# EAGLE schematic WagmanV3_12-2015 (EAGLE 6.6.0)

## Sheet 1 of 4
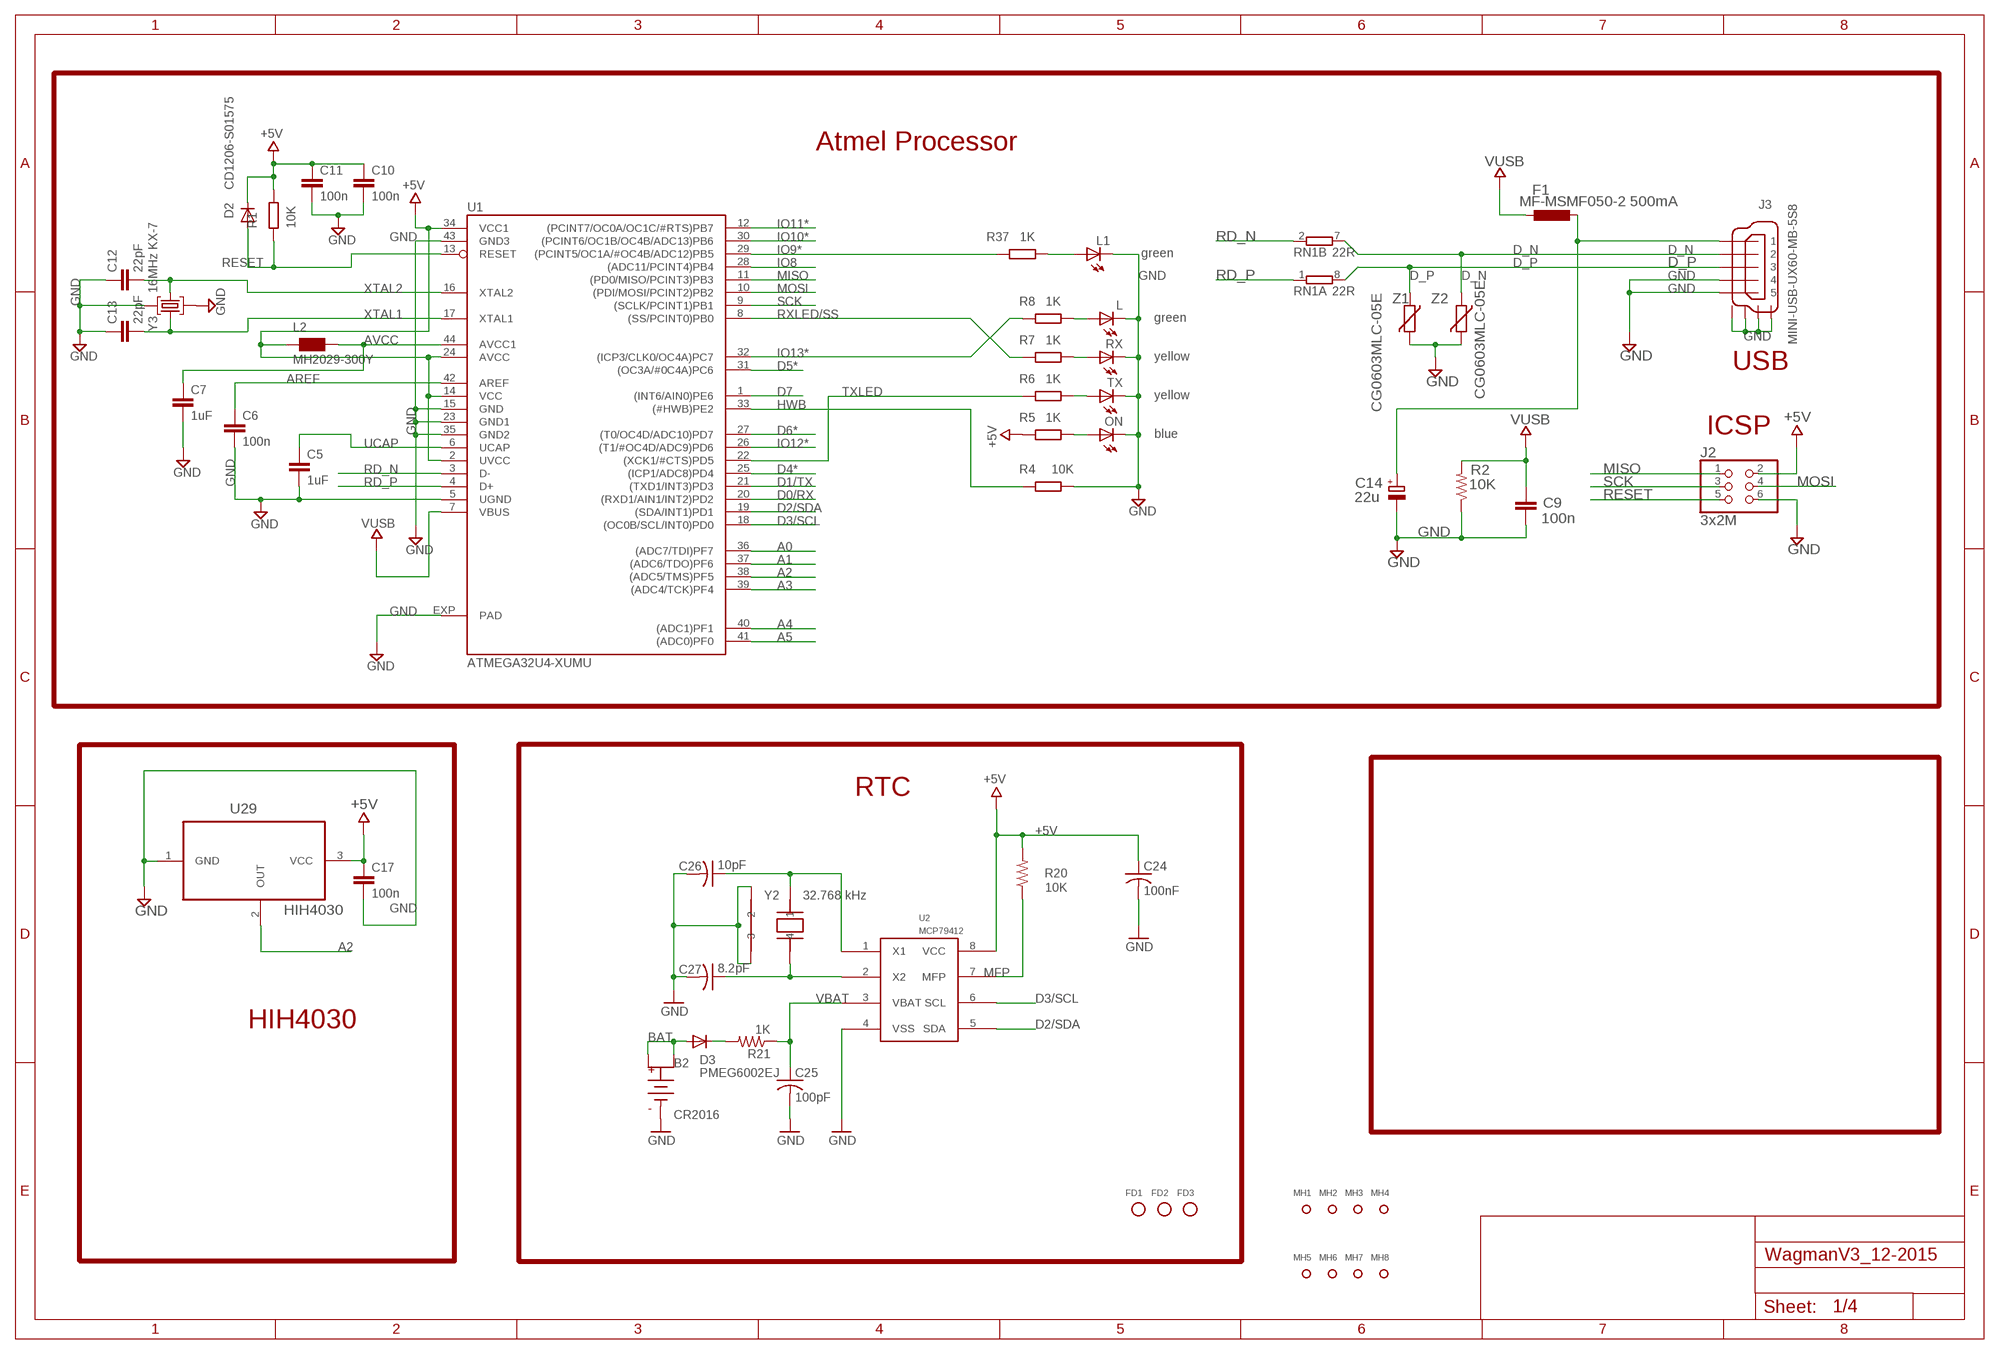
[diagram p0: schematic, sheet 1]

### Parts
B2  CR2016  COIN-CELL-2016-SMT  [BAT-HLD-002-SMT]
C5  1uF  C-EUC0402  [C0402]
C6  100n  C-EUC0402  [C0402]
C7  1uF  C-EUC0402  [C0402]
C9  100n  C-EU0805  [0805]
C10  100n  C-EUC0402  [C0402]
C11  100n  C-EUC0402  [C0402]
C12  22pF  C-EUC0402  [C0402]
C13  22pF  C-EUC0402  [C0402]
C14  22u  CPOL-EUSMCB  [SMC_B]
C17  100n  C-EUC0402  [C0402]
C24  100nF  C-USM0805  [M0805]
C25  100pF  C-USM0805  [M0805]
C26  10pF  C-USM0805  [M0805]
C27  8.2pF  C-USM0805  [M0805]
D2  CD1206-S01575  DIODE-MINIMELF  [MINIMELF]
D3  PMEG6002EJ  DIODESOD-323F  [SOD-323F]
F1  MF-MSMF050-2 500mA  L-EUL1812  [L1812]
FD1  FIDUCIAL-1MM  [FD-1MM]
FD2  FIDUCIAL-1MM  [FD-1MM]
FD3  FIDUCIAL-1MM  [FD-1MM]
J2  3x2M  PINHD-2X3  [2X03]
J3  MINI-USB-UX60-MB-5S8  [UX60-MB-5S8]
L  green  LEDCHIPLED_0805  [CHIPLED_0805]
L1  green  LEDCHIPLED_0805  [CHIPLED_0805]
L2  MH2029-300Y  WE-CBF_0805  [0805]
MH1  MH-3.964  [MH3.964]
MH2  MH-3.964  [MH3.964]
MH3  MH-3.964  [MH3.964]
MH4  MH-3.964  [MH3.964]
MH5  MH-3.964  [MH3.964]
MH6  MH-3.964  [MH3.964]
MH7  MH-3.964  [MH3.964]
MH8  MH-3.964  [MH3.964]
ON  blue  LEDCHIPLED_0805  [CHIPLED_0805]
R1  10K  R-EU_R0402  [R0402]
R2  10K  RESISTOR0805-RES  [0805]
R4  10K  R-EU_R0402  [R0402]
R5  1K  R-EU_R0402  [R0402]
R6  1K  R-EU_R0402  [R0402]
R7  1K  R-EU_R0402  [R0402]
R8  1K  R-EU_R0402  [R0402]
R20  10K  R-US_M0805  [M0805]
R21  1K  R-US_M0805  [M0805]
R37  1K  R-EU_R0402  [R0402]
RN1  22R  4R-NCAY16  [CAY16]
RX  yellow  LEDCHIPLED_0805  [CHIPLED_0805]
TX  yellow  LEDCHIPLED_0805  [CHIPLED_0805]
U1  ATMEGA32U4-XUMU  [QFN44ML7X7]
U2  MCP79412  MCP7941X-SOIC-8  [SO08]
U29  HIH4030  [HIH4030]
Y2  32.768 kHz  CRYSTAL-CITIZEN-CM2XXC  [CRYSTAL-CITIZEN-CM2XXC]
Y3  16MHz KX-7  CRYSTAL-3.2-2.5  [CRYSTAL-3.2-2.5]
Z1  CG0603MLC-05E  VARISTORCN0603  [CT/CN0603]
Z2  CG0603MLC-05E  VARISTORCN0603  [CT/CN0603]

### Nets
+5V: C10.1 C11.1 C17.1 C24.1 D2.C J2.2 L2.1 R1.1 R5.1 R20.2 U1.2(UVCC) U1.14(VCC) U1.24(AVCC) U1.34(VCC1) U2.8(VCC) U29.3(VCC) ; also sheet 2,3,4
A0: U1.36((ADC7/TDI)PF7) ; also sheet 4
A1: U1.37((ADC6/TDO)PF6) ; also sheet 4
A2: U1.38((ADC5/TMS)PF5) U29.2(OUT)
A3: U1.39((ADC4/TCK)PF4) ; also sheet 4
A4: U1.40((ADC1)PF1) ; also sheet 4
A5: U1.41((ADC0)PF0) ; also sheet 4
AREF: C6.1 U1.42(AREF)
AVCC: C7.1 L2.2 U1.44(AVCC1)
BAT: B2.POS1 B2.POS2 D3.A
D0/RX: U1.20((RXD1/AIN1/INT2)PD2) ; also sheet 3
D1/TX: U1.21((TXD1/INT3)PD3) ; also sheet 3
D2/SDA: U1.19((SDA/INT1)PD1) U2.5(SDA) ; also sheet 3
D3/SCL: U1.18((OC0B/SCL/INT0)PD0) U2.6(SCL) ; also sheet 3
D4*: U1.25((ICP1/ADC8)PD4) ; also sheet 3,4
D5*: U1.31((OC3A/#0C4A)PC6) ; also sheet 3
D6*: U1.27((T0/OC4D/ADC10)PD7) ; also sheet 3,4
D7: U1.1((INT6/AIN0)PE6) ; also sheet 4
D_N: J3.2 RN1.7 Z2.1
D_P: J3.3 RN1.8 Z1.1
GND: B2.NEG(B-) C5.2 C6.2 C7.2 C9.2 C10.2 C11.2 C12.1 C13.1 C14.- C17.2 C24.2 C25.2 C26.2 C27.2 J2.6 J3.4 J3.5 J3.M1 J3.M2 J3.M3 J3.M4 L1.C L.C ON.C R2.1 R4.2 RX.C TX.C U1.5(UGND) U1.15(GND) U1.23(GND1) U1.35(GND2) U1.43(GND3) U1.EXP(PAD) U2.4(VSS) U29.1(GND) Y2.P$2 Y2.P$3 Y3.2(GND) Y3.4(GND) Z1.2 Z2.2 ; also sheet 2,3,4
HWB: R4.1 U1.33((#HWB)PE2)
IO8: U1.28((ADC11/PCINT4)PB4) ; also sheet 3,4
IO9*: R37.1 U1.29((PCINT5/OC1A/#OC4B/ADC12)PB5)
IO10*: U1.30((PCINT6/OC1B/OC4B/ADC13)PB6) ; also sheet 3,4
IO11*: U1.12((PCINT7/OC0A/OC1C/#RTS)PB7) ; also sheet 4
IO12*: U1.26((T1/#OC4D/ADC9)PD6) ; also sheet 3,4
IO13*: R8.1 U1.32((ICP3/CLK0/OC4A)PC7)
MFP: R20.1 U2.7(MFP)
MISO: J2.1 U1.11((PD0/MISO/PCINT3)PB3)
MOSI: J2.4 U1.10((PDI/MOSI/PCINT2)PB2)
N$2: R7.2 RX.A
N$3: ON.A R5.2
N$4: R6.2 TX.A
N$7: L.A R8.2
N$15: C27.1 U2.2(X2) Y2.P$4
N$17: C26.1 U2.1(X1) Y2.P$1
N$21: D3.K R21.2
N$25: L1.A R37.2
RD_N: RN1.2 U1.3(D-)
RD_P: RN1.1 U1.4(D+)
RESET: D2.A J2.5 R1.2 U1.13(RESET)
RXLED/SS: R7.1 U1.8((SS/PCINT0)PB0)
SCK: J2.3 U1.9((SCLK/PCINT1)PB1)
TXLED: R6.1 U1.22((XCK1/#CTS)PD5)
UCAP: C5.1 U1.6(UCAP)
VBAT: C25.1 R21.1 U2.3(VBAT)
VUSB: C9.1 F1.2 R2.2 U1.7(VBUS)
VUSBD: C14.+ F1.1 J3.1
XTAL1: C13.2 U1.17(XTAL1) Y3.3(C2)
XTAL2: C12.2 U1.16(XTAL2) Y3.1(C1)
Unconnected: FD1.1 FD2.1 FD3.1 MH1.1 MH2.1 MH3.1 MH4.1 MH5.1 MH6.1 MH7.1 MH8.1 RN1.3 RN1.4 RN1.5 RN1.6

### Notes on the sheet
- Atmel Processor
- USB
- ICSP
- RTC
- HIH4030

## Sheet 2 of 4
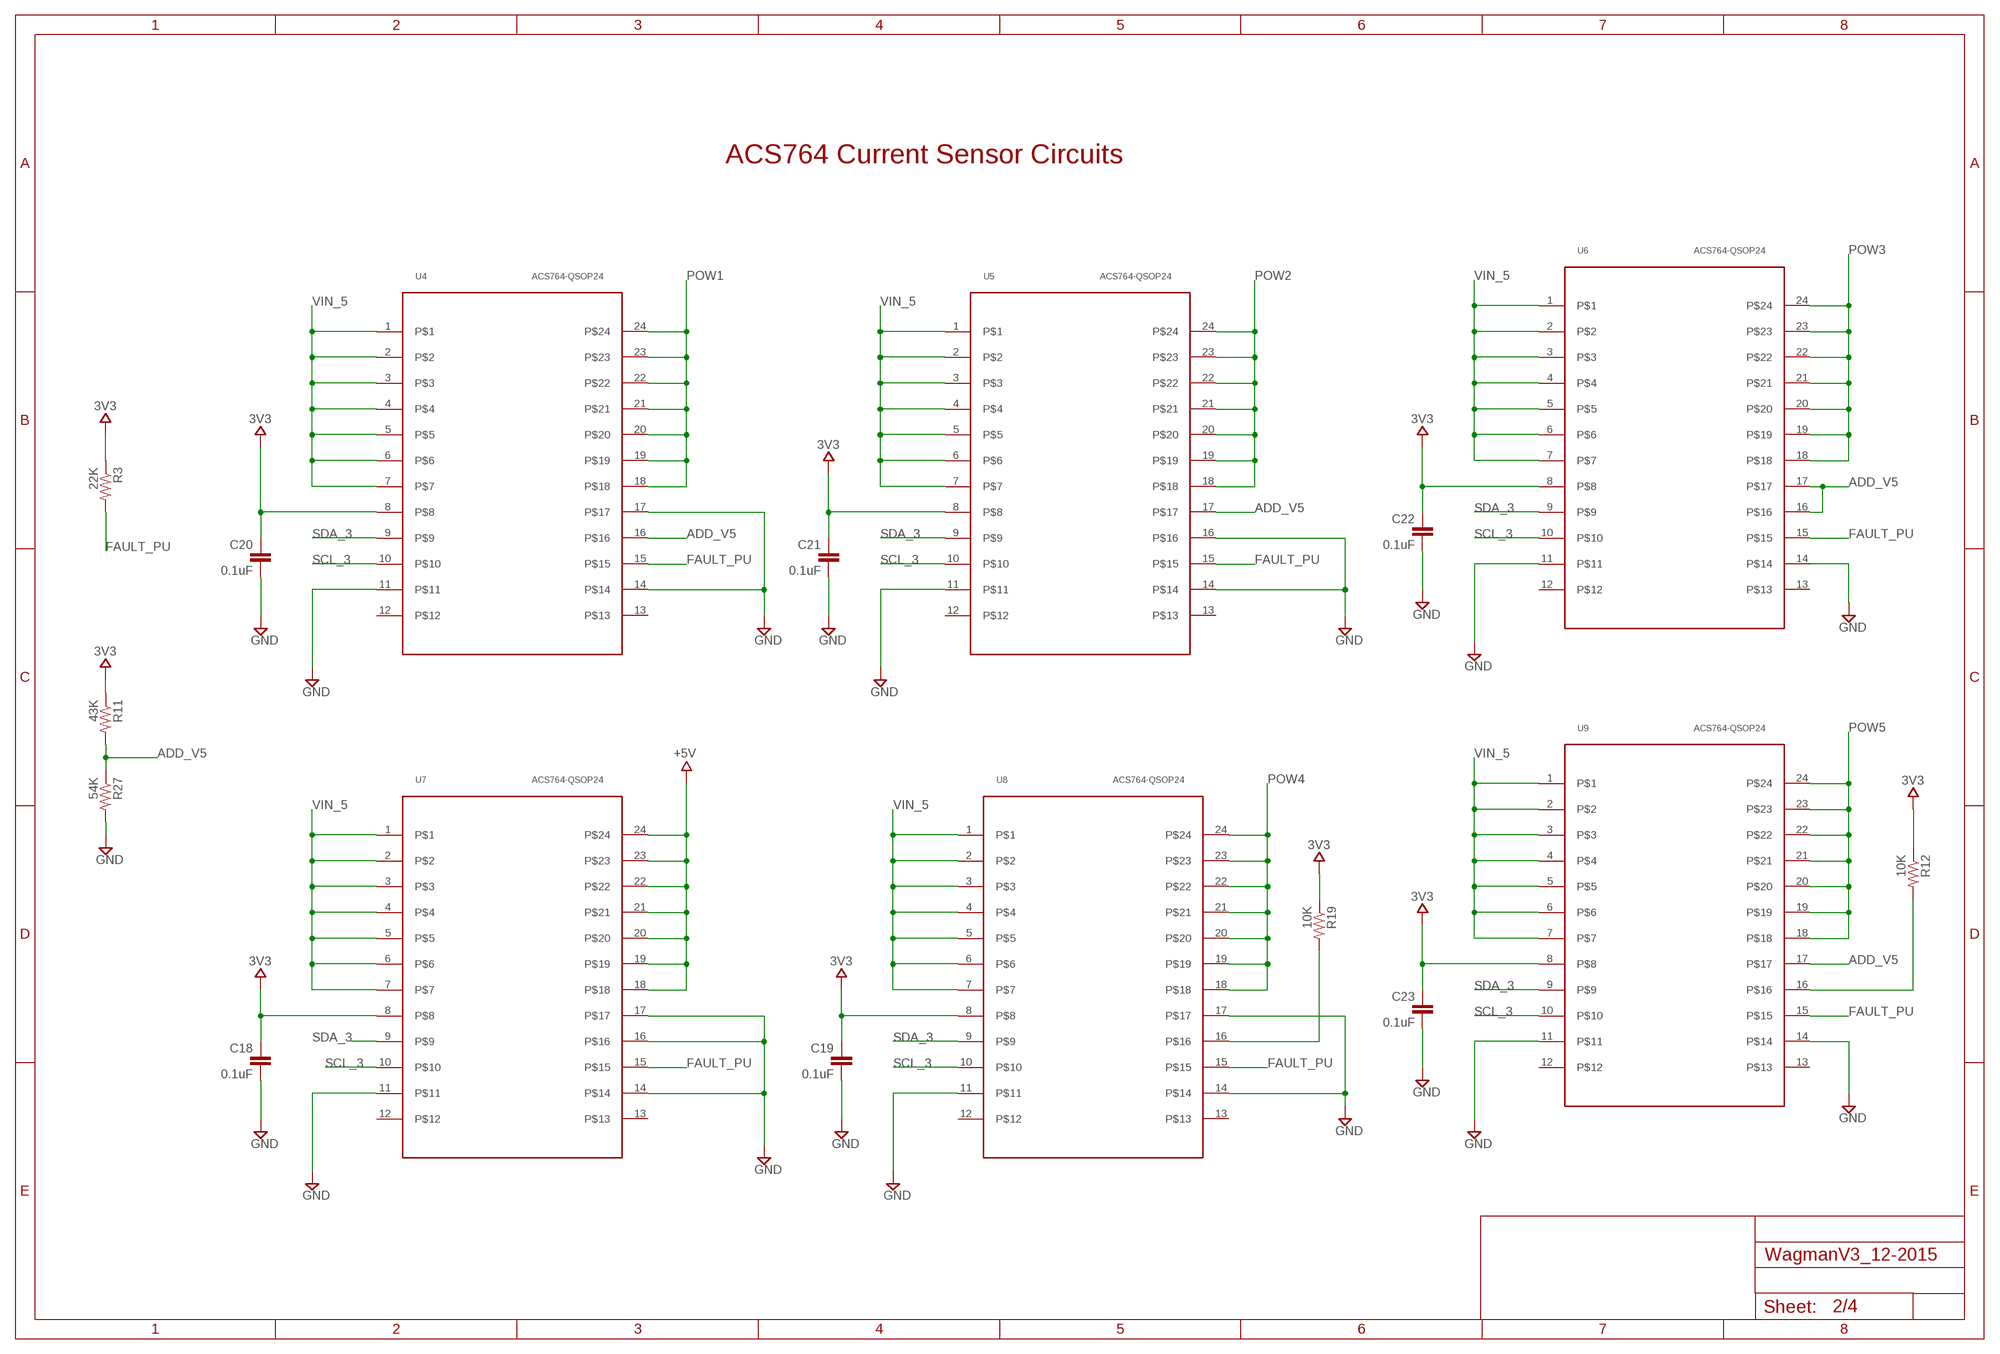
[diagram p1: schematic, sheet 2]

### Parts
C18  0.1uF  C-EUC0402  [C0402]
C19  0.1uF  C-EUC0402  [C0402]
C20  0.1uF  C-EUC0402  [C0402]
C21  0.1uF  C-EUC0402  [C0402]
C22  0.1uF  C-EUC0402  [C0402]
C23  0.1uF  C-EUC0402  [C0402]
R3  22K  RESISTOR0603-RES  [0603-RES]
R11  43K  RESISTOR0603-RES  [0603-RES]
R12  10K  RESISTOR0603-RES  [0603-RES]
R19  10K  RESISTOR0603-RES  [0603-RES]
R27  54K  RESISTOR0603-RES  [0603-RES]
U4  ACS764-QSOP24  [QSOP24]
U5  ACS764-QSOP24  [QSOP24]
U6  ACS764-QSOP24  [QSOP24]
U7  ACS764-QSOP24  [QSOP24]
U8  ACS764-QSOP24  [QSOP24]
U9  ACS764-QSOP24  [QSOP24]

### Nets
3V3: C18.1 C19.1 C20.1 C21.1 C22.1 C23.1 R3.1 R11.1 R12.1 R19.1 U4.8 U5.8 U6.8 U7.8 U8.8 U9.8 ; also sheet 3,4
+5V: U7.18 U7.19 U7.20 U7.21 U7.22 U7.23 U7.24 ; also sheet 1,3,4
ADD_V5: R11.2 R27.1 U4.16 U5.17 U6.16 U6.17 U9.17
FAULT_PU: R3.2 U4.15 U5.15 U6.15 U7.15 U8.15 U9.15
GND: C18.2 C19.2 C20.2 C21.2 C22.2 C23.2 R27.2 U4.11 U4.14 U4.17 U5.11 U5.14 U5.16 U6.11 U6.14 U7.11 U7.14 U7.16 U7.17 U8.11 U8.14 U8.17 U9.11 U9.14 ; also sheet 1,3,4
N$1: R19.2 U8.16
N$5: R12.2 U9.16
POW1: U4.18 U4.19 U4.20 U4.21 U4.22 U4.23 U4.24 ; also sheet 3
POW2: U5.18 U5.19 U5.20 U5.21 U5.22 U5.23 U5.24 ; also sheet 3
POW3: U6.18 U6.19 U6.20 U6.21 U6.22 U6.23 U6.24 ; also sheet 3
POW4: U8.18 U8.19 U8.20 U8.21 U8.22 U8.23 U8.24 ; also sheet 3
POW5: U9.18 U9.19 U9.20 U9.21 U9.22 U9.23 U9.24 ; also sheet 3
SCL_3: U4.10 U5.10 U6.10 U7.10 U8.10 U9.10 ; also sheet 3,4
SDA_3: U4.9 U5.9 U6.9 U7.9 U8.9 U9.9 ; also sheet 3,4
VIN_5: U4.1 U4.2 U4.3 U4.4 U4.5 U4.6 U4.7 U5.1 U5.2 U5.3 U5.4 U5.5 U5.6 U5.7 U6.1 U6.2 U6.3 U6.4 U6.5 U6.6 U6.7 U7.1 U7.2 U7.3 U7.4 U7.5 U7.6 U7.7 U8.1 U8.2 U8.3 U8.4 U8.5 U8.6 U8.7 U9.1 U9.2 U9.3 U9.4 U9.5 U9.6 U9.7 ; also sheet 3,4
Unconnected: U4.12 U4.13 U5.12 U5.13 U6.12 U6.13 U7.12 U7.13 U8.12 U8.13 U9.12 U9.13

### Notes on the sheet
- ACS764 Current Sensor Circuits

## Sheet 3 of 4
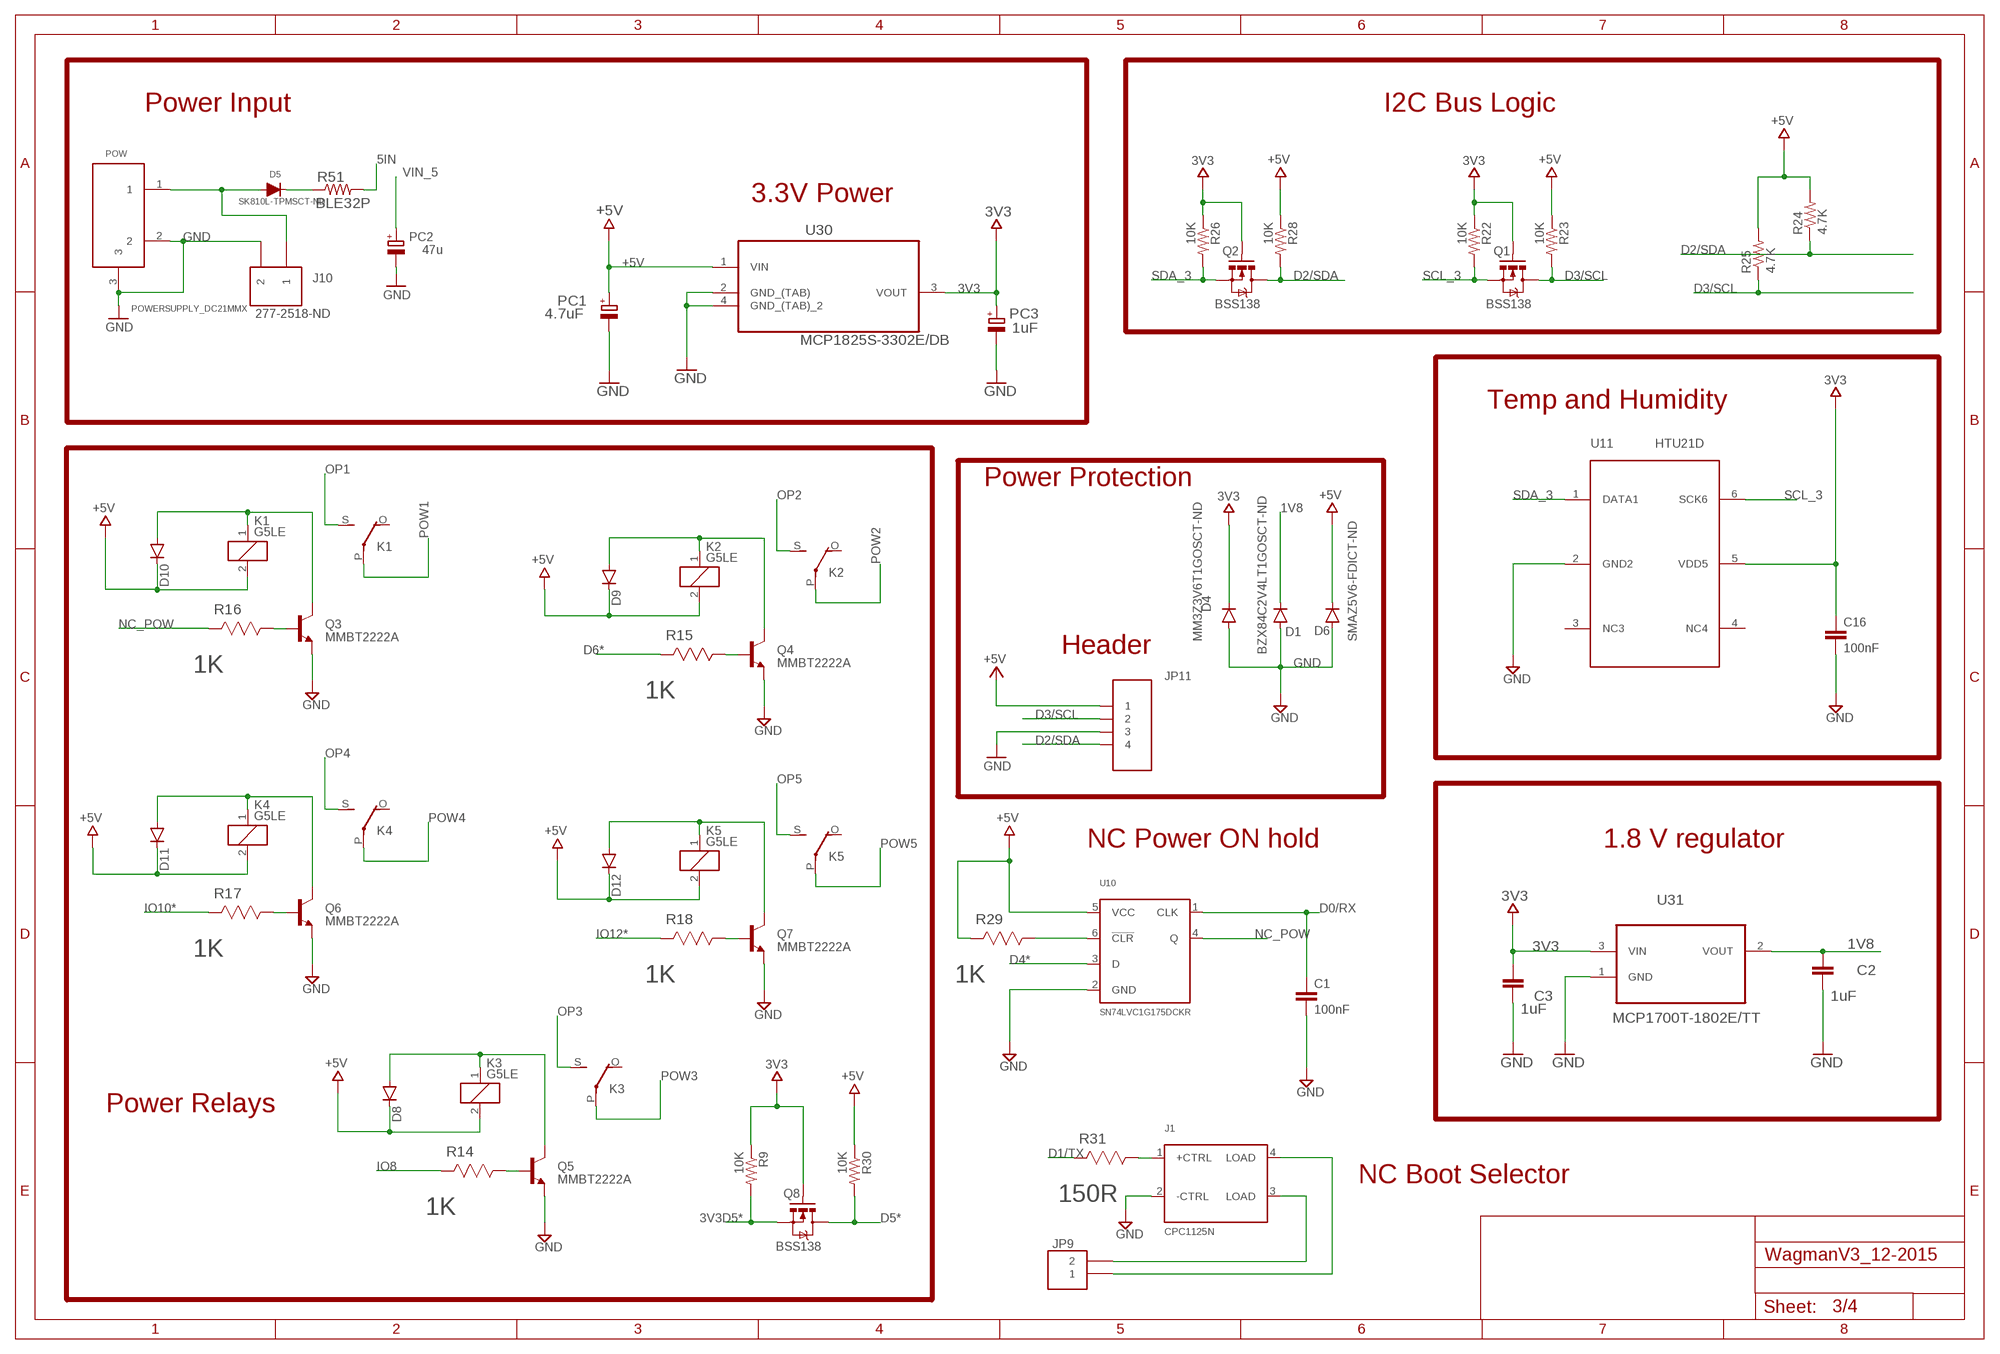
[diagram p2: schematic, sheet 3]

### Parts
C1  100nF  CAP0603-CAP  [0603-CAP]
C2  1uF  CAP0805  [0805]
C3  1uF  CAP0805  [0805]
C16  100nF  CAP0603-CAP  [0603-CAP]
D1  BZX84C2V4LT1GOSCT-ND  DIODESOT23  [SOT23-3]
D4  MM3Z3V6T1GOSCT-ND  DIODEBAS16  [SOD-323]
D5  SK810L-TPMSCT-ND  DIODEDO-214AB  [DO-214AB]
D6  SMAZ5V6-FDICT-ND  DIODESMA  [SMA-DIODE]
D8  DIODESMA  [SMA-DIODE]
D9  DIODESMA  [SMA-DIODE]
D10  DIODESMA  [SMA-DIODE]
D11  DIODESMA  [SMA-DIODE]
D12  DIODESMA  [SMA-DIODE]
J1  CPC1125N  [SOP-4]
J10  277-2518-ND  TB2-5MM  [TB2-5MM]
JP9  CONN_2PINCONN_2PIN_P2.54MM  [CONN_2PIN_P2.54MM]
JP11  147721-3  [147721-3]
K1  G5LE  [G5LE]
K2  G5LE  [G5LE]
K3  G5LE  [G5LE]
K4  G5LE  [G5LE]
K5  G5LE  [G5LE]
PC1  4.7uF  CPOL-EUD  [PANASONIC_D]
PC2  47u  CPOL-EUD  [PANASONIC_D]
PC3  1uF  CPOL-EUD  [PANASONIC_D]
POW  POWERSUPPLY_DC21MMX  [POWERSUPPLY_DC-21MM]
Q1  BSS138  MOSFET-NCHANNELSMD  [SOT23-3]
Q2  BSS138  MOSFET-NCHANNELSMD  [SOT23-3]
Q3  MMBT2222A  TRANSISTOR_NPNMMBT2222A  [SOT23-3]
Q4  MMBT2222A  TRANSISTOR_NPNMMBT2222A  [SOT23-3]
Q5  MMBT2222A  TRANSISTOR_NPNMMBT2222A  [SOT23-3]
Q6  MMBT2222A  TRANSISTOR_NPNMMBT2222A  [SOT23-3]
Q7  MMBT2222A  TRANSISTOR_NPNMMBT2222A  [SOT23-3]
Q8  BSS138  MOSFET-NCHANNELSMD  [SOT23-3]
R9  10K  RESISTOR0603-RES  [0603-RES]
R14  1K  CRM0805-FW-R050ELF  [RESC2013X65N]
R15  1K  CRM0805-FW-R050ELF  [RESC2013X65N]
R16  1K  CRM0805-FW-R050ELF  [RESC2013X65N]
R17  1K  CRM0805-FW-R050ELF  [RESC2013X65N]
R18  1K  CRM0805-FW-R050ELF  [RESC2013X65N]
R22  10K  RESISTOR0603-RES  [0603-RES]
R23  10K  RESISTOR0603-RES  [0603-RES]
R24  4.7K  4.7KOHM-1/10W-1%(0603)  [0603-RES]
R25  4.7K  4.7KOHM-1/10W-1%(0603)  [0603-RES]
R26  10K  RESISTOR0603-RES  [0603-RES]
R28  10K  RESISTOR0603-RES  [0603-RES]
R29  1K  CRM0805-FW-R050ELF  [RESC2013X65N]
R30  10K  RESISTOR0603-RES  [0603-RES]
R31  150R  CRM0805-FW-R050ELF  [RESC2013X65N]
R51  BLE32P  R-US_R1210  [R1210]
U10  SN74LVC1G175DCKR  [SOT-363]
U11  HTU21D  [DD8-3X3MM]
U30  MCP1825S-3302E/DB  [SOT230P700X180-4N]
U31  MCP1700T-1802E/TT  [SOT95P237X112-3N]

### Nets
1V8: C2.1 D1.3(C) U31.2(VOUT) ; also sheet 4
3V3: C3.1 C16.1 D4.C PC3.+ Q1.1(G) Q2.1(G) Q8.1(G) R9.1 R22.1 R26.1 U11.5(VDD5) U30.3(VOUT) U31.3(VIN) ; also sheet 2,4
3V3D5*: Q8.2(S) R9.2 ; also sheet 4
5IN: R51.2 ; also sheet 4
+5V: D6.C D8.C D9.C D10.C D11.C D12.C JP11.1 K1.2 K2.2 K3.2 K4.2 K5.2 PC1.+ R23.1 R24.2 R25.2 R28.1 R29.2(R2) R30.1 U10.5(VCC) U30.1(VIN) ; also sheet 1,2,4
D0/RX: C1.1 U10.1(CLK) ; also sheet 1
D1/TX: R31.2(R2) ; also sheet 1
D2/SDA: JP11.4 Q2.3(D) R24.1 R28.2 ; also sheet 1
D3/SCL: JP11.2 Q1.3(D) R23.2 R25.1 ; also sheet 1
D4*: U10.3(D) ; also sheet 1,4
D5*: Q8.3(D) R30.2 ; also sheet 1
D6*: R15.2(R2) ; also sheet 1,4
GND: C1.2 C2.2 C3.2 C16.2 D1.1(A) D4.A D6.A J1.2(-CTRL) J10.2 JP11.3 PC1.- PC2.- PC3.- POW.2 POW.3 Q3.2(E) Q4.2(E) Q5.2(E) Q6.2(E) Q7.2(E) U10.2(GND) U11.2(GND2) U30.2(GND_(TAB)) U30.4(GND_(TAB)_2) U31.1(GND) ; also sheet 1,2,4
IO8: R14.2(R2) ; also sheet 1,4
IO10*: R17.2(R2) ; also sheet 1,4
IO12*: R18.2(R2) ; also sheet 1,4
N$6: J1.3(LOAD) JP9.2
N$11: D8.A K3.1 Q5.3(C)
N$14: Q5.1(B) R14.1(R1)
N$16: D9.A K2.1 Q4.3(C) ; also sheet 4
N$18: Q4.1(B) R15.1(R1)
N$19: D5.A J10.1 POW.1
N$20: D10.A K1.1 Q3.3(C)
N$22: Q3.1(B) R16.1(R1)
N$23: J1.4(LOAD) JP9.1
N$24: D11.A K4.1 Q6.3(C)
N$26: Q6.1(B) R17.1(R1)
N$27: R29.1(R1) U10.6(!CLR)
N$28: D12.A K5.1 Q7.3(C)
N$30: Q7.1(B) R18.1(R1)
N$40: J1.1(+CTRL) R31.1(R1)
N$45: D5.C R51.1
NC_POW: R16.2(R2) U10.4(Q)
OP1: K1.S(2:S) ; also sheet 4
OP2: K2.S(2:S) ; also sheet 4
OP3: K3.S(2:S) ; also sheet 4
OP4: K4.S(2:S) ; also sheet 4
OP5: K5.S(2:S) ; also sheet 4
POW1: K1.P(2:P) ; also sheet 2
POW2: K2.P(2:P) ; also sheet 2
POW3: K3.P(2:P) ; also sheet 2
POW4: K4.P(2:P) ; also sheet 2
POW5: K5.P(2:P) ; also sheet 2
SCL_3: Q1.2(S) R22.2 U11.6(SCK6) ; also sheet 2,4
SDA_3: Q2.2(S) R26.2 U11.1(DATA1) ; also sheet 2,4
VIN_5: PC2.+ ; also sheet 2,4
Unconnected: K1.O(2:O) K2.O(2:O) K3.O(2:O) K4.O(2:O) K5.O(2:O) U11.3(NC3) U11.4(NC4)

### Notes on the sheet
- Power Input | I2C Bus Logic
- 3.3V Power
- Temp and Humidity
- Power Protection
- Header
- NC Power ON hold | 1.8 V regulator
- Power Relays
- NC Boot Selector

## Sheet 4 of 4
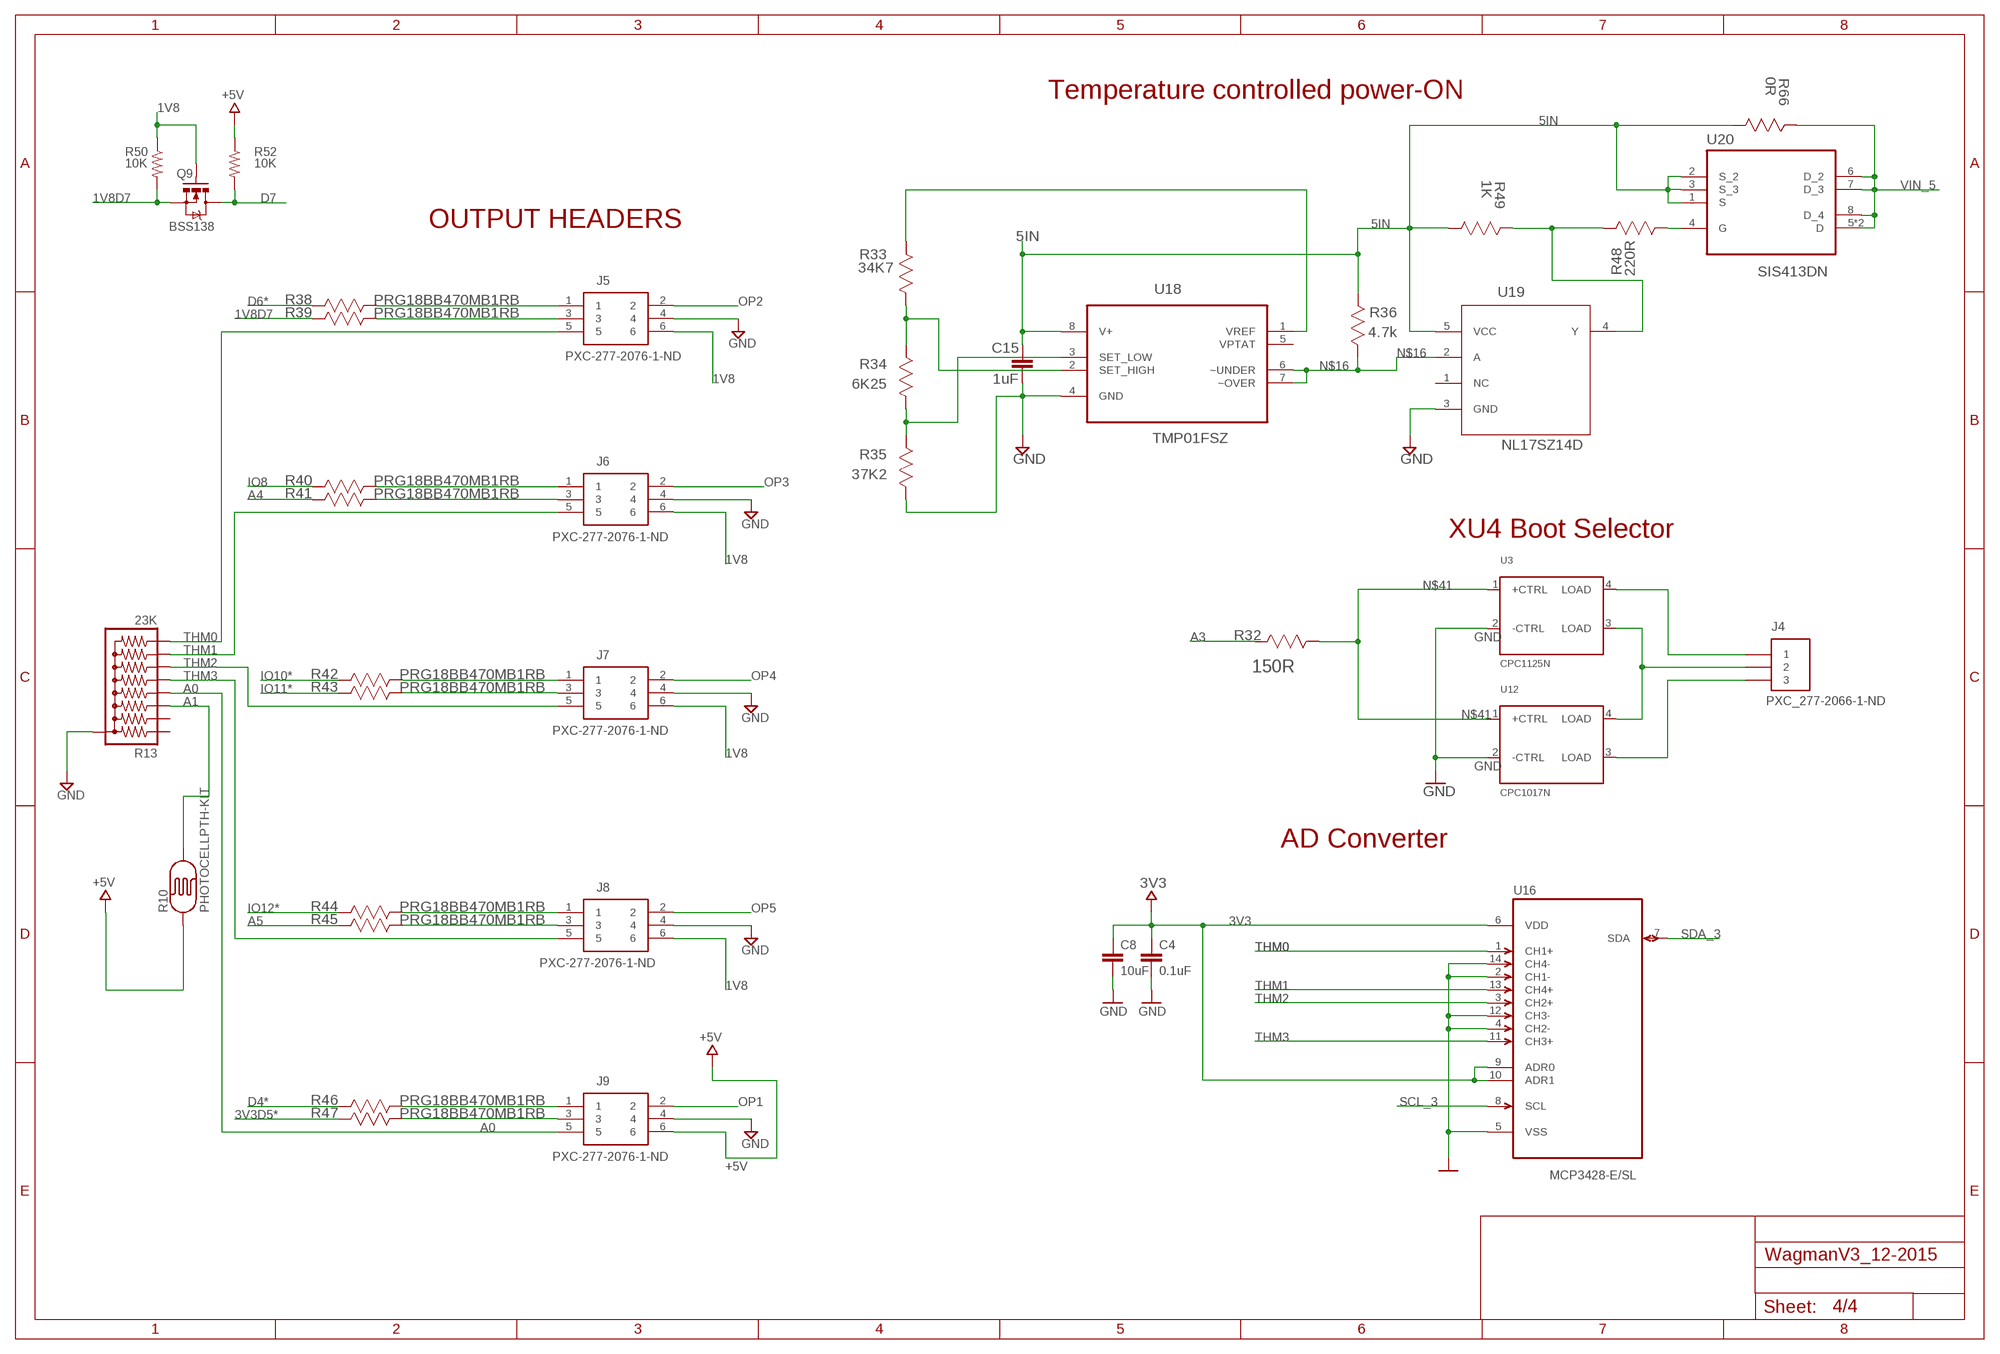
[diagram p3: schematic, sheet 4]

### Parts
C4  0.1uF  CAP0805  [0805]
C8  10uF  CAP0805  [0805]
C15  1uF  CAP0805  [0805]
J4  PXC_277-2066-1-ND  [3PIN-PTSM-RA-2.5MM]
J5  PXC-277-2076-1-ND  [6PIN-PTSM-2.5MM]
J6  PXC-277-2076-1-ND  [6PIN-PTSM-2.5MM]
J7  PXC-277-2076-1-ND  [6PIN-PTSM-2.5MM]
J8  PXC-277-2076-1-ND  [6PIN-PTSM-2.5MM]
J9  PXC-277-2076-1-ND  [6PIN-PTSM-2.5MM]
Q9  BSS138  MOSFET-NCHANNELSMD  [SOT23-3]
R10  PHOTOCELLPTH-KIT  [PHOTOCELL-KIT]
R13  23K  RPACK-BUSSED-8SIP-PTH-8-LP  [RPACK-SIP-PTH-8-LP]
R32  150R  CRM0805-FW-R050ELF  [RESC2013X65N]
R33  34K7  CRM0805-FW-R050ELF  [0805]
R34  6K25  CRM0805-FW-R050ELF  [0805]
R35  37K2  CRM0805-FW-R050ELF  [0805]
R36  4.7k  CRM0805-FW-R050ELF  [0805]
R38  PRG18BB470MB1RB  PTC-SMD  [PTC-0603]
R39  PRG18BB470MB1RB  PTC-SMD  [PTC-0603]
R40  PRG18BB470MB1RB  PTC-SMD  [PTC-0603]
R41  PRG18BB470MB1RB  PTC-SMD  [PTC-0603]
R42  PRG18BB470MB1RB  PTC-SMD  [PTC-0603]
R43  PRG18BB470MB1RB  PTC-SMD  [PTC-0603]
R44  PRG18BB470MB1RB  PTC-SMD  [PTC-0603]
R45  PRG18BB470MB1RB  PTC-SMD  [PTC-0603]
R46  PRG18BB470MB1RB  PTC-SMD  [PTC-0603]
R47  PRG18BB470MB1RB  PTC-SMD  [PTC-0603]
R48  220R  CRM0805-FW-R050ELF  [0805]
R49  1K  CRM0805-FW-R050ELF  [0805]
R50  10K  RESISTOR0603-RES  [0603-RES]
R52  10K  RESISTOR0603-RES  [0603-RES]
R66  0R  CRM0805-FW-R050ELF  [0805]
U3  CPC1125N  [SOP-4]
U12  CPC1017N  CPC1125N  [SOP-4]
U16  MCP3428-E/SL  [SOIC127P600X175-14N]
U18  TMP01FSZ  [SOIC127P600X175-8N]
U19  NL17SZ14D  74AHCT1G04W5-7  [SOT-353]
U20  SIS413DN  [SIS413]

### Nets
1V8: J5.6 J6.6 J7.6 J8.6 Q9.1(G) R50.1 ; also sheet 3
1V8D7: Q9.2(S) R39.2(R2) R50.2
3V3: C4.1 C8.1 U16.6(VDD) U16.9(ADR0) U16.10(ADR1) ; also sheet 2,3
3V3D5*: R47.2(R2) ; also sheet 3
5IN: C15.1 R36.2(R2) R49.1(R1) R66.1(R1) U18.8(V+) U19.5(VCC) U20.1(S) U20.2(S_2) U20.3(S_3) ; also sheet 3
+5V: J9.6 R10.1 R52.1 ; also sheet 1,2,3
A0: J9.5 R13.P$5 ; also sheet 1
A1: R10.2 R13.P$4 ; also sheet 1
A3: R32.2(R2) ; also sheet 1
A4: R41.2(R2) ; also sheet 1
A5: R45.2(R2) ; also sheet 1
D4*: R46.2(R2) ; also sheet 1,3
D6*: R38.2(R2) ; also sheet 1,3
D7: Q9.3(D) R52.2 ; also sheet 1
GND: C4.2 C8.2 C15.2 J5.4 J6.4 J7.4 J8.4 J9.4 R13.P$1 R35.1(R1) U3.2(-CTRL) U12.2(-CTRL) U16.2(CH1-) U16.4(CH2-) U16.5(VSS) U16.12(CH3-) U16.14(CH4-) U18.4(GND) U19.3(GND) ; also sheet 1,2,3
IO8: R40.2(R2) ; also sheet 1,3
IO10*: R42.2(R2) ; also sheet 1,3
IO11*: R43.2(R2) ; also sheet 1
IO12*: R44.2(R2) ; also sheet 1,3
N$8: R33.1(R1) R34.2(R2) U18.2(SET_HIGH)
N$9: R34.1(R1) R35.2(R2) U18.3(SET_LOW)
N$10: R33.2(R2) U18.1(VREF)
N$12: R48.1(R1) U20.4(G)
N$13: R48.2(R2) R49.2(R2) U19.4(Y)
N$16: R36.1(R1) U18.6(~UNDER) U18.7(~OVER) U19.2(A) ; also sheet 3
N$29: J5.1 R38.1(R1)
N$31: J5.3 R39.1(R1)
N$32: J6.1 R40.1(R1)
N$33: J6.3 R41.1(R1)
N$34: J7.1 R42.1(R1)
N$35: J7.3 R43.1(R1)
N$36: J8.1 R44.1(R1)
N$37: J8.3 R45.1(R1)
N$38: J9.1 R46.1(R1)
N$39: J9.3 R47.1(R1)
N$41: R32.1(R1) U3.1(+CTRL) U12.1(+CTRL)
N$42: J4.2 U3.3(LOAD) U12.4(LOAD)
N$43: J4.1 U3.4(LOAD)
N$44: J4.3 U12.3(LOAD)
OP1: J9.2 ; also sheet 3
OP2: J5.2 ; also sheet 3
OP3: J6.2 ; also sheet 3
OP4: J7.2 ; also sheet 3
OP5: J8.2 ; also sheet 3
SCL_3: U16.8(SCL) ; also sheet 2,3
SDA_3: U16.7(SDA) ; also sheet 2,3
THM0: J5.5 R13.P$9 U16.1(CH1+)
THM1: J6.5 R13.P$8 U16.13(CH4+)
THM2: J7.5 R13.P$7 U16.3(CH2+)
THM3: J8.5 R13.P$6 U16.11(CH3+)
VIN_5: R66.2(R2) U20.5(D) U20.6(D_2) U20.7(D_3) U20.8(D_4) U20.PAD(D) ; also sheet 2,3
Unconnected: R13.P$2 R13.P$3 U18.5(VPTAT) U19.1(NC)

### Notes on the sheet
- Temperature controlled power-ON
- OUTPUT HEADERS
- XU4 Boot Selector
- AD Converter

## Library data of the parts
B2 = _jc:COIN-CELL
C1 C4 C8 C16 = SparkFun:CAP: Capacitor
C2 C3 C15 = wagman_v2.3:CAP: Capacitor
C5-C7 C10-C13 C17-C23 = SmartPrj:C-EU: CAPACITOR, European symbol
C9 = wagman_v2.3:C-EU: CAPACITOR, European symbol
C14 PC1-PC3 = rcl:CPOL-EU: POLARIZED CAPACITOR, European symbol
C24-C27 = _jc:C-US: CAPACITOR, American symbol
D1 D6 = Wagman:DIODE: Diode
D2 = diode:DIODE-: DIODE
D3 = _jc:DIODE
D4 = Wagman:DIODE: Diode; PROD_ID: DIO-09646; VALUE: 250mA/100V
D5 = VS_Eagle:DIODE
D8-D12 = SparkFun-DiscreteSemi:DIODE: Diode
F1 = rcl:L-EU: INDUCTOR, European symbol
FD1-FD3 = touch+:FIDUCIAL-1MM
J1 U3 U12 = VS_Eagle:CPC1125N
J2 = SmartPrj:PINHD-2X3: PIN HEADER
J3 = mainBoard_V1R1:MINI-USB-: MINI USB Connector Source: http://www.hirose.co.jp/cataloge_hp/e24000019.pdf; OC_FARNELL: unknown; OC_NEWARK: unknown
J4 = VS_Eagle:PXC_277-2066-1-ND
J5-J9 = VS_Eagle:PXC-277-2076-1-ND
J10 = VS_Eagle:TB2-5MM
JP9 = VS_Eagle:CONN_2PIN
JP11 = VS_Eagle:147721-3
K1-K5 = relay:G5LE: RELAY 1 x switch, 10 A/120 V AC, 8 A/30 V DC, Omron; OC_FARNELL: unknown; OC_NEWARK: unknown
L L1 ON RX TX = led:LED: LED
L2 = wuerth-elektronik:WE-CBF: SMD EMI Suppression Ferrite Beads
MH1-MH8 = mainBoard:MH-3.964
POW = mainBoard_V2:POWERSUPPLY_DC21MM
Q1 Q2 Q8 Q9 = SparkFun:MOSFET-NCHANNEL
Q3-Q7 = SparkFun-DiscreteSemi:TRANSISTOR_NPN: Generic NPN BJT MMBT2222A - TRANS-08049 (SOT-23, 1A 40V) MPSA42 - TRANS-09116 (SOT-23, 500mA 300V) MMBT5088LT1G - TRANS-11160 (SOT-23, 50 mA 30V) BC547 - COM-08928 (TO-92 45V 100mA) (1.Collector 2.Base 3.Emitter) 2N3904 - COM-00521 (TO-92 40V 200mA) (1.Emitter 2.Base 3.Collector) P2N2222A -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; PROD_ID: TRANS-08049
R1 R4-R8 R37 = SmartPrj:R-EU_: RESISTOR, European symbol
R2 = wagman_v2.3:RESISTOR: Resistor
R3 R9 R11 R12 R19 R22 R23 R26-R28 R30 R50 R52 = SparkFun:RESISTOR: Resistor
R10 = SparkFun-Sensors:PHOTOCELL: CdS photoresistor. This is a low cost way to detect light levels. Resistance decreases with more incoming light. SparkFun SKU: SEN-09088
R13 = SparkFun-Resistors:RPACK-BUSSED-8: BOURNS 4600X/R series thick-film SIP resistor packs Height resistors bussed to a single pin (denoted by dot). datasheet SIMILAR TO: SFE parts COM-10855 (330), COM-10856 (10K)
R14-R18 R29 R31 R32 = Bourns_By_element14_Batch_1:CRM0805-FW-R050ELF: Resistor 0805; MPN: CRM0805-FW-R050ELF; OC_FARNELL: 1865234; OC_NEWARK: 17T4231; SUPPLIER: BOURNS; TOLERANCE: ±1 %; VALUE: 0.05 Ohm; WATTAGE: 0.25 W
R20 R21 = _jc:R-US_: RESISTOR, American symbol
R24 R25 = SparkFun-Resistors:4.7KOHM-1/10W-1%(0603): RES-07857; PROD_ID: RES-07857
R33-R36 R48 R49 R66 = wagman_v2.3:CRM0805-FW-R050ELF: Resistor 0805
R38-R47 = Wagman:PTC-SMD
R51 = Wagman:R-US_: RESISTOR, American symbol
RN1 = wagman_v2.3:4R-N: Array Chip Resistor Source: RS Component / Phycomp
U1 = SmartPrj:ATMEGA32U4-XU
U2 = _jc:MCP7941X
U4-U9 = SysMon:ACS764-QSOP24
U10 = VS_Eagle:SN74LVC1G175DCKR
U11 = SysMon:HTU21D
U16 = aux_board_v1r1:MCP3428-E/SL: Analog-to-Digital Converter; MPN: MCP3428-E/SL; OC_FARNELL: 1825014; OC_NEWARK: 52R9962; PACKAGE: SOIC-14; SUPPLIER: Microchip
U18 = Analog Devices_By_element14_Batch_1:TMP01FSZ: Low Power Programmable Temperature Controller; MPN: TMP01FSZ; OC_FARNELL: 1079393; OC_NEWARK: 96K2115; PACKAGE: SOIC-8; SUPPLIER: Analog Devices
U19 = WagmanV3_12-2015:74AHCT1G04W5-7: SINGLE INVERTER GATE
U20 = WagmanV3_12-2015:SIS413DN: MOSFET
U29 = wagman_v2.2:HIH4030
U30 = Microchip_By_element14_Batch_1:MCP1825S-3302E/DB: IC, LDO VOLT REG, 3.3V, 0.5A; MPN: MCP1825S-3302E/DB; OC_FARNELL: 1578404; OC_NEWARK: 26M9961; PACKAGE: SOT-223-3; SUPPLIER: Microchip
U31 = Microchip_By_element14_Batch_1:MCP1700T-1802E/TT: Low Quiescent Current LDO; MPN: MCP1700T-1802E/TT; OC_FARNELL: 1296591; OC_NEWARK: 84R5175; PACKAGE: SOT23-3; SUPPLIER: Microchip
Y2 = _jc:CRYSTAL-CITIZEN-CM2XXC
Y3 = SmartPrj:CRYSTAL-3.2-2.5
Z1 Z2 = varistor:VARISTOR: VARISTOR

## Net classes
0 default: width 0.254 mm, drill 0.61 mm, clearance 0.203 mm

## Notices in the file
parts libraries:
SparkFun-Sensors: Licensing: Creative Commons ShareAlike 4.0 International - https://creativecommons.org/licenses/by-sa/4.0
